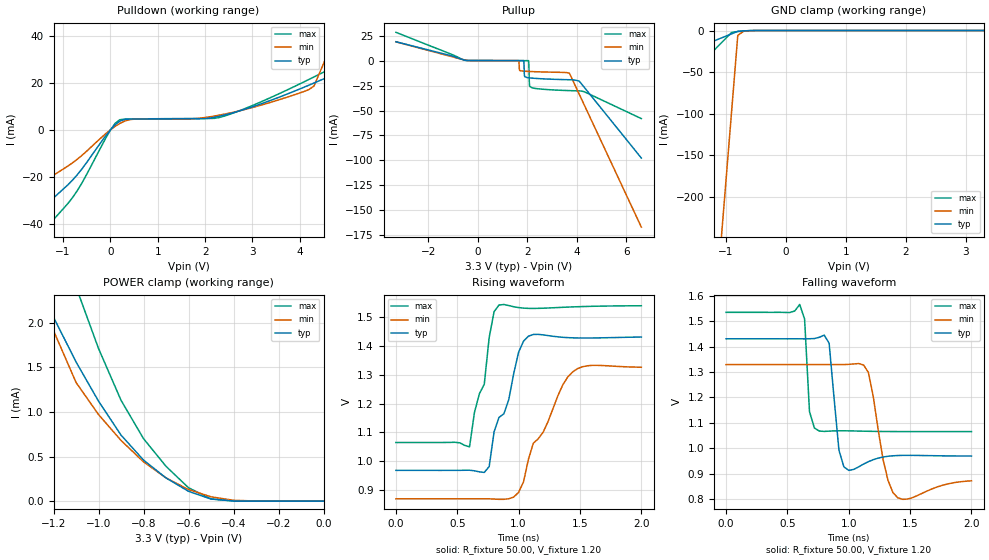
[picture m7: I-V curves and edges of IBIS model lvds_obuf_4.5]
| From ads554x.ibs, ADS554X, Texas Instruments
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|   Model lvds_obuf_4.5
[Model]   lvds_obuf_4.5
Model_type   3-state
Polarity   Non-Inverting
Enable   Active-High
Vmeas =   1.2000V
Cref =   5.0000pF
Rref = 50.0000
Vref =   1.2000V
C_comp   2.13pF   1.93pF   2.33pF
[Temperature Range]   27.00   125   -40.00
[Voltage Range]   3.30V   3.00V   3.60V
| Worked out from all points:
|   slope of the pulldown table from 0 to 0.495 V, typ, clamps not added: 107 ohm
|   GND clamp passes 1 mA (typ) near -0.79 V on its own axis
|   POWER clamp passes 1 mA (typ) near -0.97 V on its own axis
|   rising waveform, R_fixture 50.00, V_fixture 1.20: 20-80 % time 192ps typ, 271ps min, 130ps max; typ from 0.969 V to 1.43 V
|   falling waveform, R_fixture 50.00, V_fixture 1.20: 20-80 % time 52.6ps typ, 91.6ps min, 30.9ps max; typ from 1.43 V to 0.969 V
[Pulldown]
| voltage   I(typ)   I(min)   I(max)
-3.3V     -67.65mA   -46.44mA   -85.46mA
-2.1V     -45.57mA   -30.96mA   -58.46mA
-1.5V     -34.53mA   -23.22mA   -44.96mA
-800mV    -21.45mA   -14.08mA   -28.9mA
200mV     3.68mA     2.67mA     4.26mA
2.4V      6.22mA     6.6mA      5.78mA
4.3V      19.88mA    18.64mA    22.46mA
4.7V      23.52mA    37.54mA    26.48mA
4.9V      29.76mA    46.99mA    28.53mA
5.1V      48.68mA    56.44mA    30.76mA
5.5V      86.52mA    75.34mA    61.38mA
6.6V      190.6mA    127.3mA    179.9mA
[Pullup]
| voltage   I(typ)   I(min)   I(max)
-3.3V     18.97mA    18.87mA    28.41mA
-500mV    360uA      560uA      340uA
1.65V     31.69uA    10.42uA    52.57uA
1.69V     29.87uA    -9.664mA   50.23uA
1.85V     11.27uA    -10.52mA   40.84uA
1.89V     -15.63mA   -10.59mA   38.48uA
2.04V     -17.15mA   -10.8mA    28.27uA
2.06V     -17.2mA    -10.82mA   -2.019mA
2.1V      -17.3mA    -10.87mA   -25.79mA
3.7V      -19.14mA   -12.66mA   -30.03mA
4.1V      -20.66mA   -33.94mA   -30.35mA
6.6V      -97.66mA   -166.9mA   -58.1mA
[GND_clamp]
| voltage   I(typ)   I(min)   I(max)
-3.3V     -73.53mA   -2.228A    -176.7mA
-1.1V     -9.73mA    -272.6mA   -16.77mA
-1V       -6.83mA    -183.7mA   -9.5mA
-900mV    -3.93mA    -94.8mA    -2.23mA
-800mV    -1.03mA    -5.92mA    -1.19mA
-700mV    -450uA     -730uA     -490uA
3.3V      44.64pA    1.08uA     37.43pA
[POWER_clamp]
| voltage   I(typ)   I(min)   I(max)
-3.3V     247.8mA    491.9mA    558.7mA
-1.3V     2.62mA     3.21mA     3.99mA
-1.2V     2.06mA     1.91mA     3.16mA
-1.1V     1.56mA     1.33mA     2.4mA
-1V       1.12mA     970uA      1.71mA
-900mV    740uA      680uA      1.13mA
-800mV    460uA      440uA      700uA
-700mV    260uA      260uA      390uA
-600mV    110uA      130uA      150uA
-500mV    23.34uA    48.47uA    24.97uA
-400mV    2uA        9.55uA     1.31uA
0V        44.64pA    500pA      43.31pA
[Ramp]
| variable   typ   min   max
dV/dt_r   1.84/71.06p   1.61/0.12n   2.05/47.54p
dV/dt_f   1.78/0.23n   1.59/0.15n   1.83/0.30n
R_load = 1.00k
[Rising Waveform]
R_fixture = 50.00
V_fixture = 1.20
V_fixture_min = 1.10
V_fixture_max = 1.30
| time   V(typ)   V(min)   V(max)
0s        969.1mV    871mV      1.065V
600ps     969.7mV    871mV      1.05V
720ps     962mV      871mV      1.267V
760ps     982.4mV    870.8mV    1.428V
840ps     1.152V     869.1mV    1.54V
920ps     1.214V     871.2mV    1.538V
1ns       1.377V     893.4mV    1.531V
1.08ns    1.433V     1.008V     1.528V
1.44ns    1.427V     1.309V     1.534V
2ns       1.43V      1.325V     1.538V
[Falling Waveform]
R_fixture = 50.00
V_fixture = 1.20
V_fixture_min = 1.10
V_fixture_max = 1.30
| time   V(typ)   V(min)   V(max)
0s        1.431V     1.329V     1.536V
600ps     1.431V     1.329V     1.566V
640ps     1.431V     1.329V     1.509V
680ps     1.431V     1.329V     1.144V
760ps     1.437V     1.329V     1.067V
840ps     1.414V     1.329V     1.067V
960ps     926.4mV    1.329V     1.069V
1.16ns    946.7mV    1.299V     1.067V
1.4ns     971mV      804mV      1.065V
2ns       969mV      871.2mV    1.065V
